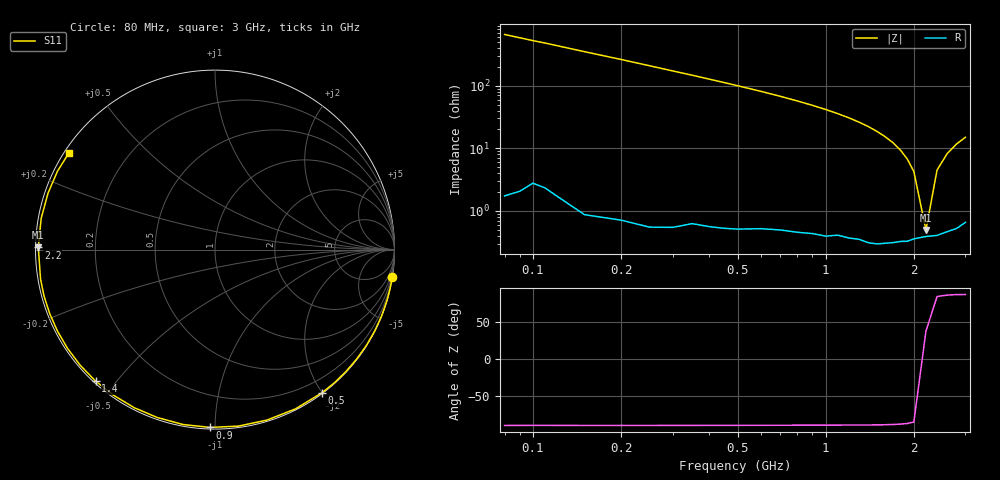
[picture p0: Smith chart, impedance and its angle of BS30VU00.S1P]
! SIEMENS Small Signal Semiconductors
! BB640
! Si Tuning Diode in SOD323
! VR = 30 V
! S-Parameters:  July  1993
# GHz  S  MA  R  50
!  f  S11
! GHz  MAG  ANG
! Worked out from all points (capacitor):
!   33 points, 80 MHz to 3 GHz, reference 50 ohm
!   read as one part to ground: C = 3.03 pF near 80 MHz
!   lowest |Z| = 496 mohm at 2.2 GHz (marker M1)
!   series resonance near 2.187 GHz, so ESL is about 1.8 nH
!   S11 on the Smith chart (normalised r, x): 80 MHz: 0, -13; 500 MHz: 0.01, -2.00; 900 MHz: 0.01, -0.97; 1.4 GHz: 0.01, -0.44; 2.2 GHz: 0.01, +0.01; 3 GHz: 0.01, +0.30
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0.08  0.9996 -8.7
0.15  0.9993 -16.3
0.2  0.999 -21.6
0.25  0.9988 -27.0
0.3  0.9983 -32.4
0.35  0.9974 -37.6
0.45  0.9965 -48.1
0.5  0.9959 -53.2
0.6  0.9943 -63.2
0.7  0.993 -73.0
0.8  0.9921 -82.5
0.9  0.9911 -91.6
1  0.9907 -100.4
1.1  0.9892 -108.9
1.2  0.9893 -117.0
1.3  0.989 -124.8
1.4  0.9897 -132.2
1.5  0.9896 -139.4
1.6  0.9889 -146.2
1.7  0.9883 -152.6
1.8  0.9875 -158.8
1.9  0.9872 -164.7
2  0.9859 -170.3
2.2  0.9845 179.3
2.4  0.984 169.8
2.6  0.982 161.3
2.8  0.9803 153.6
3  0.9762 146.6
